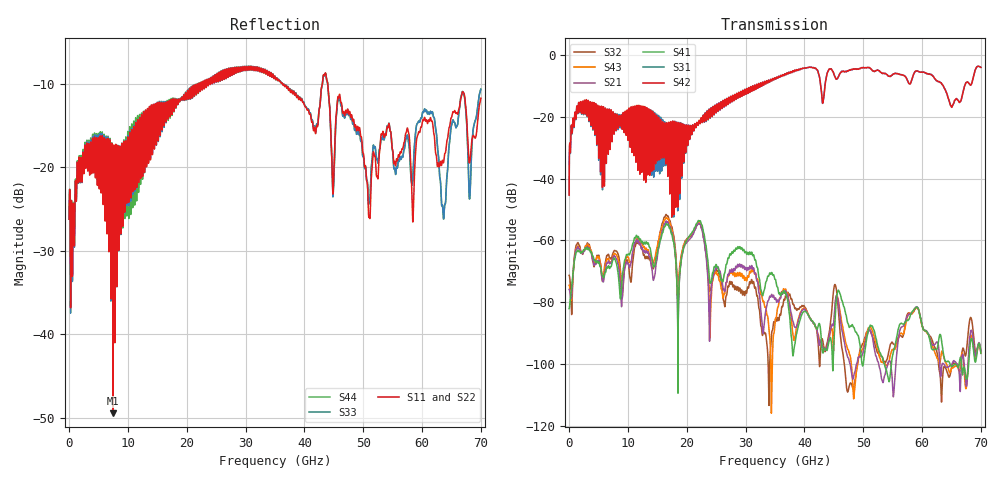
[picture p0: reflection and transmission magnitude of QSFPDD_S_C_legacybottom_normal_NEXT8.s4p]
! AWR Design Environment (8415) Thu Dec 20 14:54:15 2018
! Document = 'CHANNEL TEST'
! nPorts: 4, nXvals: 7001
# HZ S DB R 50
!Freq DBS11 AngS11 DBS12 AngS12 DBS13 AngS13 DBS14 AngS14
!	DBS21 AngS21 DBS22 AngS22 DBS23 AngS23 DBS24 AngS24
!	DBS31 AngS31 DBS32 AngS32 DBS33 AngS33 DBS34 AngS34
!	DBS41 AngS41 DBS42 AngS42 DBS43 AngS43 DBS44 AngS44
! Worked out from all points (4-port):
!   7000 points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, 10 MHz to 70 GHz, reference 50 ohm
!   strongest paths, dB at 10 MHz, 17.51 GHz, 35.01 GHz, 52.51 GHz, 70 GHz:
!     S42: -45.4, -28.7, -7.5, -5.0, -4.0
!     S31: -45.3, -28.7, -7.5, -5.0, -4.0
!     S41: -82.1, -58.1, -72.6, -94.3, -96.6
!     S21: -75.9, -57.6, -78.9, -99.2, -95.8
!     S43: -74.5, -56.8, -86.6, -95.6, -96.5
!     S32: -71.3, -55.8, -86.3, -96.5, -95.7
!   lowest |S11| = -49.4 dB at 7.45 GHz (marker M1), VSWR 1.01, Z = 50.3 + j0.0931 ohm
!   |S11| at or under -10 dB: start of sweep to 22.1 GHz; 36.25 GHz to 43.06 GHz (6.813 GHz wide, 17.2 % of centre); 43.96 GHz to end of sweep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
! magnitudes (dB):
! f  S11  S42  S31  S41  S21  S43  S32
! 10 MHz  -26.2  -45.4  -45.3  -82.1  -75.9  -74.5  -71.3
! 1.64 GHz  -19.9  -15.4  -15.5  -63.6  -62.7  -62.4  -61.4
! 7.45 GHz  -49.4  -18.5  -18.5  -66.4  -65.6  -65.3  -64.2
! 18.59 GHz  -11.9  -23.0  -22.9  -81.8  -81.8  -74.2  -78.7
! 22.09 GHz  -10.1  -21.2  -21.4  -53.7  -54.6  -54.4  -54.5
! 26.46 GHz  -8.5  -14.6  -14.6  -70.6  -76.5  -77.3  -81.5
! 70 GHz  -11.8  -4.0  -4.0  -96.6  -95.8  -96.5  -95.7
